| IBIS file 71v3578z_pf.ibs created by s2ibis2 version 1.1
| North Carolina State University Electronics Research Laboratory  1995
[IBIS ver]   2.1
[File name]   71v3578z_pf.ibs
[File Rev]   1.1
[Date]   8/11/00
[Source]   Integrated Device Technology, Inc.
[Notes]   1. Temperatures: typ=25C, min=70C, max=0C 2. Cemos10_3v
   process. 3. Ramp rates based on 50 ohm load.
[Copyright]   Copyright 2000, Integrated Device Technology, Inc. Integrated
   Device Technology, Inc. ("IDT") hereby grants the user of this
   IBIS model a non-exclusive, nontransferable license to use
   this IBIS model under the following terms. The user is granted
   this license only to use the IBIS model and is not granted
   rights to sell, copy (except as needed to run the IBIS model),
   rent, lease or sub-license the IBIS model in whole or in part,
   or in modified form to anyone. The User may modify the IBIS
   model to suit its specific applications, but rights to
   derivative works and such modifications shall belong to IDT.
   This IBIS model is provided on an AS IS" basis and IDT makes
   absolutely no warranty with respect to the information
   contained herein. IDT DISCLAIMS AND CUSTOMER WAIVES ALL
   WARRANTIES, EXPRESS AND IMPLIED, INCLUDING WARRANTIES OF
   MERCHANTABILITY AND FITNESS FOR A PARTICULAR PURPOSE. THE
   ENTIRE RISK AS TO QUALITY AND PERFORMANCE IS WITH THE USER
   ACCORDINGLY, IN NO EVENT SHALL IDT BE LIABLE FOR ANY DIRECT OR
   INDIRECT DAMAGES, WHETHER IN CONTRACT OR TORT, INCLUDING ANY
   LOST PROFITS OR OTHER INCIDENTAL, CONSEQUENTIAL, EXEMPLARY, OR
   PUNITIVE DAMAGES ARISING OUT OF THE USE OR APPLICATION OF THE
   IBIS model. Further, IDT reserves the right to make changes
   without notice to any product herein to improve reliability,
   function, or design. IDT does not convey any license under
   patent rights or any other intellectual property rights,
   including those of third parties. IDT is not obligated to
   provide maintenance or support for the licensed IBIS model.
|   Component idt71V3578Z
[Component]   idt71V3578Z
[Manufacturer]   Integrated Device Technology
|   This component uses the 100 pin TQFP package (PF)
[Package]
| variable   typ   min   max
R_pkg   0.000   0.000   0.000
L_pkg   0.000H   0.000H   0.000H
C_pkg   0.000F   0.000F   0.000F
[Pin]  signal_name   model_name   R_pin   L_pin   C_pin
1   NC   NC   6.37e-03  4.62e-09  9.13e-13
2   NC   NC   6.36e-03  4.72e-09  1.09e-12
3   NC   NC   6.49e-03  4.81e-09  1.14e-12
4   VDDQ   POWER   6.57e-03  4.90e-09  1.20e-12
5   VSS   GND   6.69e-03  4.70e-09  1.16e-12
6   NC   NC   6.36e-03  4.36e-09  1.09e-12
7   NC   NC   6.06e-03  4.05e-09  1.02e-12
8   IO8   IOPAD3578Z   5.76e-03  3.71e-09  9.52e-13
9   IO9   IOPAD3578Z   5.42e-03  3.37e-09  8.84e-13
10   VSS   GND   5.15e-03  3.07e-09  8.06e-13
11   VDDQ   POWER   4.86e-03  2.78e-09  7.49e-13
12   IO10   IOPAD3578Z   4.57e-03  2.51e-09  6.83e-13
13   IO11   IOPAD3578Z   4.27e-03  2.27e-09  6.18e-13
14   VDD   POWER   4.04e-03  2.09e-09  5.49e-13
15   VDD   POWER   3.63e-03  1.93e-09  3.51e-13
16   NC   NC   3.63e-03  1.93e-09  3.51e-13
17   VSS   GND   4.04e-03  2.09e-09  5.49e-13
18   IO12   IOPAD3578Z   4.27e-03  2.27e-09  6.18e-13
19   IO13   IOPAD3578Z   4.57e-03  2.51e-09  6.83e-13
20   VDDQ   POWER   4.86e-03  2.78e-09  7.49e-13
21   VSS   GND   5.15e-03  3.07e-09  8.06e-13
22   IO14   IOPAD3578Z   5.42e-03  3.37e-09  8.84e-13
23   IO15   IOPAD3578Z   5.76e-03  3.71e-09  9.52e-13
24   IOP2   IOPAD3578Z   6.06e-03  4.05e-09  1.02e-12
25   NC   NC   6.36e-03  4.36e-09  1.09e-12
26   VSS   GND   6.69e-03  4.70e-09  1.16e-12
27   VDDQ   POWER   6.57e-03  4.90e-09  1.20e-12
28   NC   NC   6.49e-03  4.81e-09  1.14e-12
29   NC   NC   6.36e-03  4.72e-09  1.09e-12
30   NC   NC   6.37e-03  4.62e-09  9.13e-13
31   NLBO   INPAD_71V3578Z   4.41e-03  4.16e-09  7.09e-13
32   A5   INPAD_71V3578Z   4.39e-03  4.03e-09  7.72e-13
33   A4   INPAD_71V3578Z   4.30e-03  3.88e-09  7.35e-13
34   A3   INPAD_71V3578Z   4.21e-03  3.73e-09  7.18e-13
35   A2   INPAD_71V3578Z   4.13e-03  3.60e-09  7.07e-13
36   A1   INPAD_71V3578Z   4.09e-03  3.51e-09  6.95e-13
37   A0   INPAD_71V3578Z   4.04e-03  3.41e-09  6.83e-13
38   NC   NC   3.99e-03  3.31e-09  6.74e-13
39   NC   NC   3.93e-03  3.23e-09  6.62e-13
40   VSS   GND   3.95e-03  3.18e-09  4.49e-13
41   VDD   POWER   3.95e-03  3.18e-09  4.49e-13
42   NC   NC   3.93e-03  3.23e-09  6.62e-13
43   NC   NC   3.99e-03  3.31e-09  6.74e-13
44   A11   INPAD_71V3578Z   4.04e-03  3.41e-09  6.83e-13
45   A12   INPAD_71V3578Z   4.09e-03  3.51e-09  6.95e-13
46   A13   INPAD_71V3578Z   4.13e-03  3.60e-09  7.07e-13
47   A14   INPAD_71V3578Z   4.21e-03  3.73e-09  7.18e-13
48   A15   INPAD_71V3578Z   4.30e-03  3.88e-09  7.35e-13
49   A16   INPAD_71V3578Z   4.39e-03  4.03e-09  7.72e-13
50   A17   INPAD_71V3578Z   4.41e-03  4.16e-09  7.09e-13
51   NC   NC   6.37e-03  4.62e-09  9.13e-13
52   NC   NC   6.36e-03  4.72e-09  1.09e-12
53   NC   NC   6.49e-03  4.81e-09  1.14e-12
54   VDDQ   POWER   6.57e-03  4.90e-09  1.20e-12
55   VSS   GND   6.69e-03  4.70e-09  1.16e-12
56   NC   NC   6.36e-03  4.36e-09  1.09e-12
57   NC   NC   6.06e-03  4.05e-09  1.02e-12
58   IO0   IOPAD3578Z   5.76e-03  3.71e-09  9.52e-13
59   IO1   IOPAD3578Z   5.42e-03  3.37e-09  8.84e-13
60   VSS   GND   5.15e-03  3.07e-09  8.06e-13
61   VDDQ   POWER   4.86e-03  2.78e-09  7.49e-13
62   IO2   IOPAD3578Z   4.57e-03  2.51e-09  6.83e-13
63   IO3   IOPAD3578Z   4.27e-03  2.27e-09  6.18e-13
64   ZZ   INPAD_71V3578Z   4.04e-03  2.09e-09  5.49e-13
65   VDD   POWER   3.63e-03  1.93e-09  3.51e-13
66   NC   NC   3.63e-03  1.93e-09  3.51e-13
67   VSS   GND   4.04e-03  2.09e-09  5.49e-13
68   IO4   IOPAD3578Z   4.27e-03  2.27e-09  6.18e-13
69   IO5   IOPAD3578Z   4.57e-03  2.51e-09  6.83e-13
70   VDDQ   POWER   4.86e-03  2.78e-09  7.49e-13
71   VSS   GND   5.15e-03  3.07e-09  8.06e-13
72   IO6   IOPAD3578Z   5.42e-03  3.37e-09  8.84e-13
73   IO7   IOPAD3578Z   5.76e-03  3.71e-09  9.52e-13
74   IOP1   IOPAD3578Z   6.06e-03  4.05e-09  1.02e-12
75   NC   NC   6.36e-03  4.36e-09  1.09e-12
76   VSS   GND   6.69e-03  4.70e-09  1.16e-12
77   VDDQ   POWER   6.57e-03  4.90e-09  1.20e-12
78   NC   NC   6.49e-03  4.81e-09  1.14e-12
79   NC   NC   6.36e-03  4.72e-09  1.09e-12
80   A10   INPAD_71V3578Z   6.37e-03  4.62e-09  9.13e-13
81   A9   INPAD_71V3578Z   4.41e-03  4.16e-09  7.09e-13
82   A8   INPAD_71V3578Z   4.39e-03  4.03e-09  7.72e-13
83   NADV   INPAD_71V3578Z   4.30e-03  3.88e-09  7.35e-13
84   NADSP   INPAD_71V3578Z   4.21e-03  3.73e-09  7.18e-13
85   NADSC   INPAD_71V3578Z   4.13e-03  3.60e-09  7.07e-13
86   NOE   INPAD_71V3578Z   4.09e-03  3.51e-09  6.95e-13
87   NBWE   INPAD_71V3578Z   4.04e-03  3.41e-09  6.83e-13
88   NGW   INPAD_71V3578Z   3.99e-03  3.31e-09  6.74e-13
89   CLK   INCLK_71V3578Z   3.93e-03  3.23e-09  6.62e-13
90   VSS   GND   3.95e-03  3.18e-09  4.49e-13
91   VDD   POWER   3.95e-03  3.18e-09  4.49e-13
92   NCS1   INPAD_71V3578Z   3.93e-03  3.23e-09  6.62e-13
93   NBW1   INPAD_71V3578Z   3.99e-03  3.31e-09  6.74e-13
94   NBW2   INPAD_71V3578Z   4.04e-03  3.41e-09  6.83e-13
95   NC   NC   4.09e-03  3.51e-09  6.95e-13
96   NC   NC   4.13e-03  3.60e-09  7.07e-13
97   CS0   INPAD_71V3578Z   4.21e-03  3.73e-09  7.18e-13
98   NCE   INPAD_71V3578Z   4.30e-03  3.88e-09  7.35e-13
99   A7   INPAD_71V3578Z   4.39e-03  4.03e-09  7.72e-13
100   A6   INPAD_71V3578Z   4.41e-03  4.16e-09  7.09e-13
1000   GNDQ   GND
| IOIN IOIN   dummy_model
| OC   OC   dummy_model
| IN   IN   dummy_model
| CLK  CLK   dummy_model
[Pin Mapping]  pulldown_ref   pullup_ref   gnd_clamp_ref   power_clamp_ref
1   NC   NC   NC   NC
2   NC   NC   NC   NC
3   NC   NC   NC   NC
4   NC   EXTVDDQ
5   EXTGND   NC
6   NC   NC   NC   NC
7   NC   NC   NC   NC
8   EXTGNDQ   EXTVDDQ   EXTGND   EXTVDD
9   EXTGNDQ   EXTVDDQ   EXTGND   EXTVDD
10   EXTGND   NC
11   NC   EXTVDDQ
12   EXTGNDQ   EXTVDDQ   EXTGND   EXTVDD
13   EXTGNDQ   EXTVDDQ   EXTGND   EXTVDD
14   NC   EXTVDD
15   NC   EXTVDD
16   NC   NC   NC   NC
17   EXTGND   NC
18   EXTGNDQ   EXTVDDQ   EXTGND   EXTVDD
19   EXTGNDQ   EXTVDDQ   EXTGND   EXTVDD
20   NC   EXTVDDQ
21   EXTGND   NC
22   EXTGNDQ   EXTVDDQ   EXTGND   EXTVDD
23   EXTGNDQ   EXTVDDQ   EXTGND   EXTVDD
24   EXTGNDQ   EXTVDDQ   EXTGND   EXTVDD
25   NC   NC   NC   NC
26   EXTGND   NC
27   NC   EXTVDDQ
28   NC   NC   NC   NC
29   NC   NC   NC   NC
30   NC   NC   NC   NC
31   EXTGNDQ   EXTVDDQ   EXTGND   EXTVDD
32   EXTGNDQ   EXTVDDQ   EXTGND   EXTVDD
33   EXTGNDQ   EXTVDDQ   EXTGND   EXTVDD
34   EXTGNDQ   EXTVDDQ   EXTGND   EXTVDD
35   EXTGNDQ   EXTVDDQ   EXTGND   EXTVDD
36   EXTGNDQ   EXTVDDQ   EXTGND   EXTVDD
37   EXTGNDQ   EXTVDDQ   EXTGND   EXTVDD
38   NC   NC   NC   NC
39   NC   NC   NC   NC
40   EXTGND   NC
41   NC   EXTVDD
42   NC   NC   NC   NC
43   NC   NC   NC   NC
44   EXTGNDQ   EXTVDDQ   EXTGND   EXTVDD
45   EXTGNDQ   EXTVDDQ   EXTGND   EXTVDD
46   EXTGNDQ   EXTVDDQ   EXTGND   EXTVDD
47   EXTGNDQ   EXTVDDQ   EXTGND   EXTVDD
48   EXTGNDQ   EXTVDDQ   EXTGND   EXTVDD
49   EXTGNDQ   EXTVDDQ   EXTGND   EXTVDD
50   EXTGNDQ   EXTVDDQ   EXTGND   EXTVDD
51   NC   NC   NC   NC
52   NC   NC   NC   NC
53   NC   NC   NC   NC
54   NC   EXTVDDQ
55   EXTGND   NC
56   NC   NC   NC   NC
57   NC   NC   NC   NC
58   EXTGNDQ   EXTVDDQ   EXTGND   EXTVDD
59   EXTGNDQ   EXTVDDQ   EXTGND   EXTVDD
60   EXTGND   NC
61   NC   EXTVDDQ
62   EXTGNDQ   EXTVDDQ   EXTGND   EXTVDD
63   EXTGNDQ   EXTVDDQ   EXTGND   EXTVDD
64   EXTGNDQ   EXTVDDQ   EXTGND   EXTVDD
65   NC   EXTVDD
66   NC   NC   NC   NC
67   EXTGND   NC
68   EXTGNDQ   EXTVDDQ   EXTGND   EXTVDD
69   EXTGNDQ   EXTVDDQ   EXTGND   EXTVDD
70   NC   EXTVDDQ
71   EXTGND   NC
72   EXTGNDQ   EXTVDDQ   EXTGND   EXTVDD
73   EXTGNDQ   EXTVDDQ   EXTGND   EXTVDD
74   EXTGNDQ   EXTVDDQ   EXTGND   EXTVDD
75   NC   NC   NC   NC
76   EXTGND   NC
77   NC   EXTVDDQ
78   NC   NC   NC   NC
79   NC   NC   NC   NC
80   EXTGNDQ   EXTVDDQ   EXTGND   EXTVDD
81   EXTGNDQ   EXTVDDQ   EXTGND   EXTVDD
82   EXTGNDQ   EXTVDDQ   EXTGND   EXTVDD
83   EXTGNDQ   EXTVDDQ   EXTGND   EXTVDD
84   EXTGNDQ   EXTVDDQ   EXTGND   EXTVDD
85   EXTGNDQ   EXTVDDQ   EXTGND   EXTVDD
86   EXTGNDQ   EXTVDDQ   EXTGND   EXTVDD
87   EXTGNDQ   EXTVDDQ   EXTGND   EXTVDD
88   EXTGNDQ   EXTVDDQ   EXTGND   EXTVDD
89   EXTGNDQ   EXTVDDQ   EXTGND   EXTVDD
90   EXTGND   NC
91   NC   EXTVDD
92   EXTGNDQ   EXTVDDQ   EXTGND   EXTVDD
93   EXTGNDQ   EXTVDDQ   EXTGND   EXTVDD
94   EXTGNDQ   EXTVDDQ   EXTGND   EXTVDD
95   NC   NC   NC   NC
96   NC   NC   NC   NC
97   EXTGNDQ   EXTVDDQ   EXTGND   EXTVDD
98   EXTGNDQ   EXTVDDQ   EXTGND   EXTVDD
99   EXTGNDQ   EXTVDDQ   EXTGND   EXTVDD
100   EXTGNDQ   EXTVDDQ   EXTGND   EXTVDD
1000   EXTGNDQ   NC
| Models and submodels in the file (3): IOPAD3578Z (I/O), INCLK_71V3578Z (Input), INPAD_71V3578Z (Input)
